| IBIS file stm32g031_041_ufqfpn32.ibs
[IBIS ver]   4.2
[File name]  stm32g031_041_ufqfpn32.ibs
[File Rev]   1.0
[Date]   31-05-2019
[Source]   Data Created at STMicroelectronics
[Notes]   File originated from ELDO simulations.
[Disclaimer] This information is for modeling purpose only and is
   not guaranted. The information is subject to change without
   notice.
[Copyright]  Copyright 2019 STMicroelectronics Inc.
|   Component stm32g031_041_ufqfpn32
[Component]   stm32g031_041_ufqfpn32
[Manufacturer] STMicroelectronics
[Package]
| variable   typ   min   max
R_pkg   0.0   0.0   0.0
L_pkg   0.0H   0.0H   0.0H
C_pkg   0.0F   0.0F   0.0F
[Pin]   signal_name   model_name  R_pin L_pin C_pin
1 PB9 io6_i2c_ft
2 PC14-OSC32_IN io8prog2m25m50m120m_sudq_ft
3 PC15-OSC32_OUT io8prog2m25m50m120m_sudq_ft
4 VDD/VDDA POWER
5 VSS/VSSA GND
6 PF2-NRST io6reset
7 PA0 io6_ft
8 PA1 io6_ft
9 PA2 io6_ft
10 PA3 io6_ft
11 PA4 io6_ft
12 PA5 io6_ft
13 PA6 io6_ft
14 PA7 io6_ft
15 PB0 io6_ft
16 PB1 io6_ft
17 PB2 io6_ft
18 PA8 io6_ft
19 PA9 io6_i2c_ft
20 PC6 io6_ft
21 PA10 io6_i2c_ft
22 PA11[PA9] io6_i2c_ft
23 PA12[PA10] io6_i2c_ft
24 PA13 io6_ft
25 PA14-BOOT0 io6_ft
26 PA15 io6_ft
27 PB3 io6_ft
28 PB4 io6_ft
29 PB5 io6_ft
30 PB6 io6_i2c_ft
31 PB7 io6_i2c_ft
32 PB8 io6_i2c_ft
[Model Selector] io8prog2m25m50m120m_sudq_ft
iols8p_sudq_ft_pd_lv  "IO low speed, PD=40kOhm - 1P8V"
iols8p_sudq_ft_pu_lv  "IO low speed, PU=40kOhm - 1P8V"
iols8p_sudq_ft_lv  "IO low speed - 1P8V"
iols8p_sudq_ft_pd  "IO low speed, PD=40kOhm - 3P3V"
iols8p_sudq_ft_pu  "IO low speed, PU=40kOhm - 3P3V"
iols8p_sudq_ft  "IO low speed - 3P3V"
iofs8p_sudq_ft_pd_lv  "IO full speed, PD=40kOhm - 1P8V"
iofs8p_sudq_ft_pu_lv  "IO full speed, PU=40kOhm - 1P8V"
iofs8p_sudq_ft_lv  "IO full speed - 1P8V"
iofs8p_sudq_ft_pd  "IO full speed, PD=40kOhm - 3P3V"
iofs8p_sudq_ft_pu  "IO full speed, PU=40kOhm - 3P3V"
iofs8p_sudq_ft  "IO full speed - 3P3V"
ioms8p_sudq_ft_pd_lv  "IO medium speed, PD=40kOhm - 1P8V"
ioms8p_sudq_ft_pu_lv  "IO medium speed, PU=40kOhm - 1P8V"
ioms8p_sudq_ft_lv  "IO medium speed - 1P8V"
ioms8p_sudq_ft_pd  "IO medium speed, PD=40kOhm - 3P3V"
ioms8p_sudq_ft_pu  "IO medium speed, PU=40kOhm - 3P3V"
ioms8p_sudq_ft  "IO medium speed - 3P3V"
iohs8p_sudq_ft_pd_lv  "IO high speed, PD=40kOhm - 1P8V"
iohs8p_sudq_ft_pu_lv  "IO high speed, PU=40kOhm - 1P8V"
iohs8p_sudq_ft_lv  "IO high speed - 1P8V"
iohs8p_sudq_ft_pd  "IO high speed, PD=40kOhm - 3P3V"
iohs8p_sudq_ft_pu  "IO high speed, PU=40kOhm - 3P3V"
iohs8p_sudq_ft  "IO high speed - 3P3V"
[Model Selector] io6_ft
io6_ft_1v8_highspeed_pd  "GPIO-1.8V range - high speed - pull down"
io6_ft_1v8_fastspeed_pd  "GPIO-1.8V range - fast speed - pull down"
io6_ft_1v8_mediumspeed_pd  "GPIO-1.8V range - medium speed - pull down"
io6_ft_1v8_lowspeed_pd  "GPIO-1.8V range - low speed - pull down"
io6_ft_1v8_highspeed_pu  "GPIO-1.8V range - high speed - pull up"
io6_ft_1v8_fastspeed_pu  "GPIO-1.8V range - fast speed - pull up"
io6_ft_1v8_mediumspeed_pu  "GPIO-1.8V range - medium speed - pull up"
io6_ft_1v8_lowspeed_pu  "GPIO-1.8V range - low speed - pull up"
io6_ft_1v8_highspeed  "GPIO-1.8V range - high speed"
io6_ft_1v8_fastspeed  "GPIO-1.8V range - fast speed"
io6_ft_1v8_mediumspeed  "GPIO-1.8V range - medium speed"
io6_ft_1v8_lowspeed  "GPIO-1.8V range - low speed"
io6_ft_3v3_highspeed_pd  "GPIO-3.3V range - high speed - pull down"
io6_ft_3v3_fastspeed_pd  "GPIO-3.3V range - fast speed - pull down"
io6_ft_3v3_mediumspeed_pd  "GPIO-3.3V range - medium speed - pull down"
io6_ft_3v3_lowspeed_pd  "GPIO-3.3V range - low speed - pull down"
io6_ft_3v3_highspeed_pu  "GPIO-3.3V range - high speed - pull up"
io6_ft_3v3_fastspeed_pu  "GPIO-3.3V range - fast speed - pull up"
io6_ft_3v3_mediumspeed_pu  "GPIO-3.3V range - medium speed - pull up"
io6_ft_3v3_lowspeed_pu  "GPIO-3.3V range - low speed - pull up"
io6_ft_3v3_highspeed  "GPIO-3.3V range - high speed"
io6_ft_3v3_fastspeed  "GPIO-3.3V range - fast speed"
io6_ft_3v3_mediumspeed  "GPIO-3.3V range - medium speed"
io6_ft_3v3_lowspeed  "GPIO-3.3V range - low speed"
[Model Selector] io6_i2c_ft
io6_ft_1v8_highspeed_pd  "GPIO-1.8V range - high speed - pull down"
io6_ft_1v8_fastspeed_pd  "GPIO-1.8V range - fast speed - pull down"
io6_ft_1v8_mediumspeed_pd  "GPIO-1.8V range - medium speed - pull down"
io6_ft_1v8_lowspeed_pd  "GPIO-1.8V range - low speed - pull down"
io6_ft_1v8_highspeed_pu  "GPIO-1.8V range - high speed - pull up"
io6_ft_1v8_fastspeed_pu  "GPIO-1.8V range - fast speed - pull up"
io6_ft_1v8_mediumspeed_pu  "GPIO-1.8V range - medium speed - pull up"
io6_ft_1v8_lowspeed_pu  "GPIO-1.8V range - low speed - pull up"
io6_ft_1v8_highspeed  "GPIO-1.8V range - high speed"
io6_ft_1v8_fastspeed  "GPIO-1.8V range - fast speed"
io6_ft_1v8_mediumspeed  "GPIO-1.8V range - medium speed"
io6_ft_1v8_lowspeed  "GPIO-1.8V range - low speed"
io6_ft_3v3_highspeed_pd  "GPIO-3.3V range - high speed - pull down"
io6_ft_3v3_fastspeed_pd  "GPIO-3.3V range - fast speed - pull down"
io6_ft_3v3_mediumspeed_pd  "GPIO-3.3V range - medium speed - pull down"
io6_ft_3v3_lowspeed_pd  "GPIO-3.3V range - low speed - pull down"
io6_ft_3v3_highspeed_pu  "GPIO-3.3V range - high speed - pull up"
io6_ft_3v3_fastspeed_pu  "GPIO-3.3V range - fast speed - pull up"
io6_ft_3v3_mediumspeed_pu  "GPIO-3.3V range - medium speed - pull up"
io6_ft_3v3_lowspeed_pu  "GPIO-3.3V range - low speed - pull up"
io6_ft_3v3_highspeed  "GPIO-3.3V range - high speed"
io6_ft_3v3_fastspeed  "GPIO-3.3V range - fast speed"
io6_ft_3v3_mediumspeed  "GPIO-3.3V range - medium speed"
io6_ft_3v3_lowspeed  "GPIO-3.3V range - low speed"
io6_i2c_ft_1v8_pd  "GPIO-1.8V I2C functionality - pull down"
io6_i2c_ft_3v3_pd  "GPIO-3.3V I2C functionality - pull down"
io6_i2c_ft_1v8_pu  "GPIO-1.8V I2C functionality - pull up"
io6_i2c_ft_3v3_pu  "GPIO-3.3V I2C functionality pull up"
io6_i2c_ft_1v8  "GPIO-1.8V I2C functionality"
io6_i2c_ft_3v3  "GPIO-3.3V I2C functionality"
[Model Selector] io6reset
io6_ft_1v8_highspeed_pd  "GPIO-1.8V range - high speed - pull down"
io6_ft_1v8_fastspeed_pd  "GPIO-1.8V range - fast speed - pull down"
io6_ft_1v8_mediumspeed_pd  "GPIO-1.8V range - medium speed - pull down"
io6_ft_1v8_lowspeed_pd  "GPIO-1.8V range - low speed - pull down"
io6_ft_1v8_highspeed_pu  "GPIO-1.8V range - high speed - pull up"
io6_ft_1v8_fastspeed_pu  "GPIO-1.8V range - fast speed - pull up"
io6_ft_1v8_mediumspeed_pu  "GPIO-1.8V range - medium speed - pull up"
io6_ft_1v8_lowspeed_pu  "GPIO-1.8V range - low speed - pull up"
io6_ft_1v8_highspeed  "GPIO-1.8V range - high speed"
io6_ft_1v8_fastspeed  "GPIO-1.8V range - fast speed"
io6_ft_1v8_mediumspeed  "GPIO-1.8V range - medium speed"
io6_ft_1v8_lowspeed  "GPIO-1.8V range - low speed"
io6_ft_3v3_highspeed_pd  "GPIO-3.3V range - high speed - pull down"
io6_ft_3v3_fastspeed_pd  "GPIO-3.3V range - fast speed - pull down"
io6_ft_3v3_mediumspeed_pd  "GPIO-3.3V range - medium speed - pull down"
io6_ft_3v3_lowspeed_pd  "GPIO-3.3V range - low speed - pull down"
io6_ft_3v3_highspeed_pu  "GPIO-3.3V range - high speed - pull up"
io6_ft_3v3_fastspeed_pu  "GPIO-3.3V range - fast speed - pull up"
io6_ft_3v3_mediumspeed_pu  "GPIO-3.3V range - medium speed - pull up"
io6_ft_3v3_lowspeed_pu  "GPIO-3.3V range - low speed - pull up"
io6_ft_3v3_highspeed  "GPIO-3.3V range - high speed"
io6_ft_3v3_fastspeed  "GPIO-3.3V range - fast speed"
io6_ft_3v3_mediumspeed  "GPIO-3.3V range - medium speed"
io6_ft_3v3_lowspeed  "GPIO-3.3V range - low speed"
ioreset_1v2_pu  "RESET 1.2V range with PU"
ioreset_1v2  "RESET 1.2V range"
ioreset_1v8_pu  "RESET 1.8V range with PU"
ioreset_1v8  "RESET 1.8V range"
ioreset_3v3_pu  "RESET 3.3V range with PU"
ioreset_3v3  "RESET 3.3V range"
| Models and submodels in the file (60): iols8p_sudq_ft_pd_lv (I/O), iols8p_sudq_ft_pu_lv (I/O), iols8p_sudq_ft_lv (I/O), iols8p_sudq_ft_pd (I/O), iols8p_sudq_ft_pu (I/O), iols8p_sudq_ft (I/O), iofs8p_sudq_ft_pd_lv (I/O), iofs8p_sudq_ft_pu_lv (I/O), iofs8p_sudq_ft_lv (I/O), iofs8p_sudq_ft_pd (I/O), iofs8p_sudq_ft_pu (I/O), iofs8p_sudq_ft (I/O), ioms8p_sudq_ft_pd_lv (I/O), ioms8p_sudq_ft_pu_lv (I/O), ioms8p_sudq_ft_lv (I/O), ioms8p_sudq_ft_pd (I/O), ioms8p_sudq_ft_pu (I/O), ioms8p_sudq_ft (I/O), iohs8p_sudq_ft_pd_lv (I/O), iohs8p_sudq_ft_pu_lv (I/O), iohs8p_sudq_ft_lv (I/O), iohs8p_sudq_ft_pd (I/O), iohs8p_sudq_ft_pu (I/O), iohs8p_sudq_ft (I/O), io6_ft_1v8_highspeed_pd (I/O), io6_ft_1v8_fastspeed_pd (I/O), io6_ft_1v8_mediumspeed_pd (I/O), io6_ft_1v8_lowspeed_pd (I/O), io6_ft_1v8_highspeed_pu (I/O), io6_ft_1v8_fastspeed_pu (I/O), io6_ft_1v8_mediumspeed_pu (I/O), io6_ft_1v8_lowspeed_pu (I/O), io6_ft_1v8_highspeed (I/O), io6_ft_1v8_fastspeed (I/O), io6_ft_1v8_mediumspeed (I/O), io6_ft_1v8_lowspeed (I/O), io6_ft_3v3_highspeed_pd (I/O), io6_ft_3v3_fastspeed_pd (I/O), io6_ft_3v3_mediumspeed_pd (I/O), io6_ft_3v3_lowspeed_pd (I/O), io6_ft_3v3_highspeed_pu (I/O), io6_ft_3v3_fastspeed_pu (I/O), io6_ft_3v3_mediumspeed_pu (I/O), io6_ft_3v3_lowspeed_pu (I/O), io6_ft_3v3_highspeed (I/O), io6_ft_3v3_fastspeed (I/O), io6_ft_3v3_mediumspeed (I/O), io6_ft_3v3_lowspeed (I/O), io6_i2c_ft_1v8_pd (I/O_open_drain), io6_i2c_ft_3v3_pd (I/O_open_drain), io6_i2c_ft_1v8_pu (I/O_open_drain), io6_i2c_ft_3v3_pu (I/O_open_drain), io6_i2c_ft_1v8 (I/O_open_drain), io6_i2c_ft_3v3 (I/O_open_drain), ioreset_1v2_pu (I/O_open_drain), ioreset_1v2 (I/O_open_drain), ioreset_1v8_pu (I/O_open_drain), ioreset_1v8 (I/O_open_drain), ioreset_3v3_pu (I/O_open_drain), ioreset_3v3 (I/O_open_drain)
